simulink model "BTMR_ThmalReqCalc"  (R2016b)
settings: Solver=FixedStepDiscrete  StartTime=0.0  StopTime=10.0  FixedStep=0.1  RelTol=1e-3  EnableMultiTasking=on
undefined symbols (not defined in the file or in its folder): BMS_cntThmStbNum_C, BTMR_cntThmalReqVal_C, BTMR_flgCoolPwrCal_C, BTMR_pChrgClntPwrLv1_C, BTMR_pChrgClntPwrLv2_C, BTMR_pChrgClntPwrLv3_C, BTMR_pChrgClntPwrLv4_C, BTMR_pChrgClntPwrLv5_C, BTMR_pChrgClntPwrLv6_C, BTMR_pCoolPwrVal_C, BTMR_pHtgACPwrReq_C, BTMR_pHtgDCPwrReq_C, BTMR_pHtgDrvPwrReq_C, BTMR_pHtgsStage1_CUR, BTMR_pHtgsStage2_CUR, BTMR_pNormClntPwrLv1_C, BTMR_pNormClntPwrLv2_C, BTMR_pNormClntPwrLv3_C, BTMR_r861BrsDrvSoc_C, BTMR_r861HtgDrvSoc_C, BTMR_r891BrsDrvSoc_C, BTMR_r891HtgDrvSoc_C, BTMR_rCoolClbFlg_C, BTMR_rFlashClbFlg_C, BTMR_rHeatClbFlg_C, BTMR_t861BrsDiffLv0Temp_C, BTMR_t861BrsDiffLv1Temp_C, BTMR_t861CoolChrgAces2Temp_C, BTMR_t861CoolChrgAces3Temp_C, BTMR_t861CoolChrgAcesTemp_C, BTMR_t861CoolChrgDiffDebTemp_C, BTMR_t861CoolChrgEndDiffTemp_C, BTMR_t861CoolChrgExitLv2Temp_C, BTMR_t861CoolChrgExitLv3Temp_C, BTMR_t861CoolChrgExitTemp_C, BTMR_t861CoolChrgIntLv0Temp_C, BTMR_t861CoolChrgIntLv1Temp_C, BTMR_t861CoolChrgIntLv2Temp_C, BTMR_t861CoolChrgIntLv3Temp_C, BTMR_t861CoolChrgIntLv4Temp_C, BTMR_t861CoolChrgIntLv5Temp_C, BTMR_t861CoolDCDebTemp_C, BTMR_t861CoolNormAcesTemp_C, BTMR_t861CoolNormDiffDebTemp_C, BTMR_t861CoolNormEndDiffTemp_C, BTMR_t861CoolNormExitLv2Temp_C, BTMR_t861CoolNormExitLv3Temp_C, BTMR_t861CoolNormExitTemp_C, BTMR_t861CoolNormIntLv0Temp_C, BTMR_t861CoolNormIntLv1Temp_C, BTMR_t861CoolNormLv2Temp_C, BTMR_t861CoolNormLv3Temp_C, BTMR_t861HtgACDiffDebTemp_C, BTMR_t861HtgACEndDiffTemp_C, BTMR_t861HtgACStartHiTemp_C, BTMR_t861HtgACStartLoTemp_C, BTMR_t861HtgACStopTemp_C, BTMR_t861HtgDCDiffDebTemp_C, BTMR_t861HtgDCEndDiffTemp_C, BTMR_t861HtgDCIntLv0Temp_C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
libraries: AIWAYS_Powertrain_BMS_lib x78, simulink x9
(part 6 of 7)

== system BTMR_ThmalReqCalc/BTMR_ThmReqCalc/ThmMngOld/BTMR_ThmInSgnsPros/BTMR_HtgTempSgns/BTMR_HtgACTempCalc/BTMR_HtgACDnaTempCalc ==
  BSPR_tCellTempMin : Inport
  BMSDebounceStartZero : AIWAYS_Powertrain_BMS_lib/Debounce & Delay/BMSDebounceStartZero
  Constant29 : Constant  Value=BTMR_tiTempBase_C
  Constant30 : Constant  Value=BTMR_tiTempDebs_C
  Constant8 : Constant  Value=BTMR_t861HtgACStopTemp_C
  Relational Operator18 : RelationalOperator  OutDataTypeStr=boolean  RndMeth=Simplest
  BTMR_flgHtgACDnaTemp : Outport
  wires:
  Constant8/1 -> Relational Operator18/2
  BMSDebounceStartZero/1 -> BTMR_flgHtgACDnaTemp/1
  Relational Operator18/1 -> BMSDebounceStartZero/1
  BSPR_tCellTempMin/1 -> Relational Operator18/1
  Constant29/1 -> BMSDebounceStartZero/5, BMSDebounceStartZero/3
  Constant30/1 -> BMSDebounceStartZero/4, BMSDebounceStartZero/2

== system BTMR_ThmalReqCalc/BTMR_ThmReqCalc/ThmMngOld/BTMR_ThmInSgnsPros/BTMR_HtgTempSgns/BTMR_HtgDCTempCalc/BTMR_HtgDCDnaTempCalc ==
  BSPR_tCellTempMin : Inport
  BSPR_tCellTempMax : Inport  Port=2
  BMSDebounceStartZero : AIWAYS_Powertrain_BMS_lib/Debounce & Delay/BMSDebounceStartZero
  Constant1 : Constant  Value=BTMR_t861HtgDCStopTemp2_C
  Constant16 : Constant  Value=BTMR_t861HtgDCStopTemp_C
  Constant29 : Constant  Value=BTMR_tiTempBase_C
  Constant30 : Constant  Value=BTMR_tiTempDebs_C
  Logical Operator4 : Logic  Operator=OR  AllPortsSameDT=off  OutDataTypeStr=boolean
  Relational Operator1 : RelationalOperator  Operator=>  OutDataTypeStr=boolean  RndMeth=Simplest
  Relational Operator18 : RelationalOperator  Operator=>  OutDataTypeStr=boolean  RndMeth=Simplest
  BTMR_flgHtgDCDnaTemp : Outport
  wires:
  BSPR_tCellTempMin/1 -> Relational Operator18/1
  Relational Operator18/1 -> Logical Operator4/1
  BMSDebounceStartZero/1 -> BTMR_flgHtgDCDnaTemp/1
  Constant16/1 -> Relational Operator18/2
  BSPR_tCellTempMax/1 -> Relational Operator1/1
  Constant1/1 -> Relational Operator1/2
  Relational Operator1/1 -> Logical Operator4/2
  Logical Operator4/1 -> BMSDebounceStartZero/1
  Constant29/1 -> BMSDebounceStartZero/5, BMSDebounceStartZero/3
  Constant30/1 -> BMSDebounceStartZero/4, BMSDebounceStartZero/2

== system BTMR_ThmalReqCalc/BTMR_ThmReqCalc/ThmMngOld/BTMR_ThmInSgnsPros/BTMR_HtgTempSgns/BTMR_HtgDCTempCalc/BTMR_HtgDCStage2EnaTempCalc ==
  BSPR_tClntUsT : Inport
  BMSDebounceStartZero : AIWAYS_Powertrain_BMS_lib/Debounce & Delay/BMSDebounceStartZero
  Constant22 : Constant  Value=BTMR_t861HtgDCIntLv4Temp_C
  Constant29 : Constant  Value=BTMR_tiTempBase_C
  Constant30 : Constant  Value=BTMR_tiTempDebs_C
  Relational Operator20 : RelationalOperator  OutDataTypeStr=boolean  RndMeth=Simplest
  BTMR_flgHtgDCStage2EnaTemp : Outport
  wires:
  BSPR_tClntUsT/1 -> Relational Operator20/1
  BMSDebounceStartZero/1 -> BTMR_flgHtgDCStage2EnaTemp/1
  Relational Operator20/1 -> BMSDebounceStartZero/1
  Constant22/1 -> Relational Operator20/2
  Constant29/1 -> BMSDebounceStartZero/5, BMSDebounceStartZero/3
  Constant30/1 -> BMSDebounceStartZero/4, BMSDebounceStartZero/2

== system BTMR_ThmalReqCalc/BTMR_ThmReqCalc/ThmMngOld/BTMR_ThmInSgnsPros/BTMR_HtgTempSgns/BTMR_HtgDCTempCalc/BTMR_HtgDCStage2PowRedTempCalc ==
  BSPR_tClntUsT : Inport
  BMSDebounceStartZero : AIWAYS_Powertrain_BMS_lib/Debounce & Delay/BMSDebounceStartZero
  Constant22 : Constant  Value=BTMR_t861HtgDCIntLv3Temp_C
  Constant29 : Constant  Value=BTMR_tiTempBase_C
  Constant30 : Constant  Value=BTMR_tiTempDebs_C
  Relational Operator20 : RelationalOperator  OutDataTypeStr=boolean  RndMeth=Simplest
  BTMR_flgHtgDCStage2PowRedTemp : Outport
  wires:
  Constant22/1 -> Relational Operator20/2
  Relational Operator20/1 -> BMSDebounceStartZero/1
  BMSDebounceStartZero/1 -> BTMR_flgHtgDCStage2PowRedTemp/1
  BSPR_tClntUsT/1 -> Relational Operator20/1
  Constant29/1 -> BMSDebounceStartZero/5, BMSDebounceStartZero/3
  Constant30/1 -> BMSDebounceStartZero/4, BMSDebounceStartZero/2

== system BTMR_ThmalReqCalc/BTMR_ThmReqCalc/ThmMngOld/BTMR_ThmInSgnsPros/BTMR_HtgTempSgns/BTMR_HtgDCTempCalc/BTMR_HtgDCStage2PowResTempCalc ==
  BSPR_tClntUsT : Inport
  BMSDebounceStartZero : AIWAYS_Powertrain_BMS_lib/Debounce & Delay/BMSDebounceStartZero
  Constant22 : Constant  Value=BTMR_t861HtgDCIntLv2Temp_C
  Constant29 : Constant  Value=BTMR_tiTempBase_C
  Constant30 : Constant  Value=BTMR_tiTempDebs_C
  Relational Operator20 : RelationalOperator  Operator=<=  OutDataTypeStr=boolean  RndMeth=Simplest
  BTMR_flgHtgDCStage2PowResTemp : Outport
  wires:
  BSPR_tClntUsT/1 -> Relational Operator20/1
  BMSDebounceStartZero/1 -> BTMR_flgHtgDCStage2PowResTemp/1
  Relational Operator20/1 -> BMSDebounceStartZero/1
  Constant22/1 -> Relational Operator20/2
  Constant29/1 -> BMSDebounceStartZero/5, BMSDebounceStartZero/3
  Constant30/1 -> BMSDebounceStartZero/4, BMSDebounceStartZero/2

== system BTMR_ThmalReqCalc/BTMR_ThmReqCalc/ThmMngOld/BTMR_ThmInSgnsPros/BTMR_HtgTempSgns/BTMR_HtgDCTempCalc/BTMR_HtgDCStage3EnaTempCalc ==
  BSPR_tCellTempMin : Inport
  BSPR_tCellTempMax : Inport  Port=2
  BMSDebounceStartZero : AIWAYS_Powertrain_BMS_lib/Debounce & Delay/BMSDebounceStartZero
  Constant23 : Constant  Value=BTMR_t861HtgDCStageMxTemp_C
  Constant24 : Constant  Value=BTMR_t861HtgDCStageMnTemp_C
  Constant29 : Constant  Value=BTMR_tiTempBase_C
  Constant30 : Constant  Value=BTMR_tiTempDebs_C
  Logical Operator1 : Logic  Operator=NOT  AllPortsSameDT=off  OutDataTypeStr=boolean
  Logical Operator4 : Logic  AllPortsSameDT=off  OutDataTypeStr=boolean
  Relational Operator12 : RelationalOperator  Operator=<  OutDataTypeStr=boolean  RndMeth=Simplest
  Relational Operator13 : RelationalOperator  Operator=<  OutDataTypeStr=boolean  RndMeth=Simplest
  BTMR_flgHtgDCStage3EnaTemp : Outport
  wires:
  BSPR_tCellTempMin/1 -> Relational Operator12/1
  Logical Operator4/1 -> Logical Operator1/1
  Constant24/1 -> Relational Operator12/2
  Relational Operator13/1 -> Logical Operator4/2
  Constant23/1 -> Relational Operator13/2
  Relational Operator12/1 -> Logical Operator4/1
  BMSDebounceStartZero/1 -> BTMR_flgHtgDCStage3EnaTemp/1
  BSPR_tCellTempMax/1 -> Relational Operator13/1
  Logical Operator1/1 -> BMSDebounceStartZero/1
  Constant29/1 -> BMSDebounceStartZero/5, BMSDebounceStartZero/3
  Constant30/1 -> BMSDebounceStartZero/4, BMSDebounceStartZero/2

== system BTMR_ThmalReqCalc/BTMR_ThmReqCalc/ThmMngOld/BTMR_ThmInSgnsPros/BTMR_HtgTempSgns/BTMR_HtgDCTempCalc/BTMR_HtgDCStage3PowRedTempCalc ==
  BSPR_tClntUsT : Inport
  BMSDebounceStartZero : AIWAYS_Powertrain_BMS_lib/Debounce & Delay/BMSDebounceStartZero
  Constant22 : Constant  Value=BTMR_t861HtgDCIntLv1Temp_C
  Constant29 : Constant  Value=BTMR_tiTempBase_C
  Constant30 : Constant  Value=BTMR_tiTempDebs_C
  Relational Operator20 : RelationalOperator  Operator=<=  OutDataTypeStr=boolean  RndMeth=Simplest
  BTMR_flgHtgDCStage3PowRedTemp : Outport
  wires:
  BSPR_tClntUsT/1 -> Relational Operator20/1
  BMSDebounceStartZero/1 -> BTMR_flgHtgDCStage3PowRedTemp/1
  Relational Operator20/1 -> BMSDebounceStartZero/1
  Constant22/1 -> Relational Operator20/2
  Constant29/1 -> BMSDebounceStartZero/5, BMSDebounceStartZero/3
  Constant30/1 -> BMSDebounceStartZero/4, BMSDebounceStartZero/2

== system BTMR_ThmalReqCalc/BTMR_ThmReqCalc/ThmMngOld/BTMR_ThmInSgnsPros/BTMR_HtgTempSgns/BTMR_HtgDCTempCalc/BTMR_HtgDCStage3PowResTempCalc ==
  BSPR_tClntUsT : Inport
  BMSDebounceStartZero : AIWAYS_Powertrain_BMS_lib/Debounce & Delay/BMSDebounceStartZero
  Constant22 : Constant  Value=BTMR_t861HtgDCIntLv0Temp_C
  Constant29 : Constant  Value=BTMR_tiTempBase_C
  Constant30 : Constant  Value=BTMR_tiTempDebs_C
  Relational Operator20 : RelationalOperator  Operator=<=  OutDataTypeStr=boolean  RndMeth=Simplest
  BTMR_flgHtgDCStage3PowResTemp : Outport
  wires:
  Constant22/1 -> Relational Operator20/2
  Relational Operator20/1 -> BMSDebounceStartZero/1
  BMSDebounceStartZero/1 -> BTMR_flgHtgDCStage3PowResTemp/1
  BSPR_tClntUsT/1 -> Relational Operator20/1
  Constant29/1 -> BMSDebounceStartZero/5, BMSDebounceStartZero/3
  Constant30/1 -> BMSDebounceStartZero/4, BMSDebounceStartZero/2

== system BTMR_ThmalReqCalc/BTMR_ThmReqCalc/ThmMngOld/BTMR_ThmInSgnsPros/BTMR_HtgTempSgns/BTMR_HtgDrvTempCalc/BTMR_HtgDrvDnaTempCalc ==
  BSPR_tCellTempMin : Inport
  BMSDebounceStartZero : AIWAYS_Powertrain_BMS_lib/Debounce & Delay/BMSDebounceStartZero
  Constant2 : Constant  Value=BTMR_t861HtgDrvStopTemp_C
  Constant29 : Constant  Value=BTMR_tiTempBase_C
  Constant30 : Constant  Value=BTMR_tiTempDebs_C
  Relational Operator18 : RelationalOperator  OutDataTypeStr=boolean  RndMeth=Simplest
  BTMR_flgHtgDrvDnaTemp : Outport
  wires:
  BSPR_tCellTempMin/1 -> Relational Operator18/1
  Relational Operator18/1 -> BMSDebounceStartZero/1
  BMSDebounceStartZero/1 -> BTMR_flgHtgDrvDnaTemp/1
  Constant2/1 -> Relational Operator18/2
  Constant29/1 -> BMSDebounceStartZero/5, BMSDebounceStartZero/3
  Constant30/1 -> BMSDebounceStartZero/4, BMSDebounceStartZero/2

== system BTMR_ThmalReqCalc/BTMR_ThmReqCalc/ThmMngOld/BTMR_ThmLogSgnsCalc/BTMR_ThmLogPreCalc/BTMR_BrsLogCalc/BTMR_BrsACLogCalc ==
  BTMR_flgBMSStsSgns : Inport
  BTMR_flgBrsEnSgns : Inport  Port=2
  BTMR_flgBrsIntSgns : Inport  Port=3
  Bus Creator : BusCreator  Inputs=3
  Bus Selector : BusSelector  OutputSignals=BTMR_flgBMSAChrg
  Bus Selector2 : BusSelector  OutputSignals=BTMR_flgBrsEna2Temp
  Bus Selector3 : BusSelector  OutputSignals=BTMR_flgBrsIntEna2Temp
  Logical Operator1 : Logic  Operator=NOT  AllPortsSameDT=off  OutDataTypeStr=boolean
  Logical Operator{2..4,6} (4 alike) : Logic  AllPortsSameDT=off  OutDataTypeStr=boolean
  Logical Operator5 : Logic  Operator=NOT  AllPortsSameDT=off  OutDataTypeStr=boolean
  BTMR_flgBrsACLogSgns : Outport
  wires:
  Bus Selector3/1 -> Logical Operator5/1, Logical Operator3/2  "<BTMR_flgBrsIntEna2Temp>"
  Logical Operator6/1 -> Logical Operator3/1, Logical Operator4/1  "BTMR_flgBrsEna2"
  Logical Operator2/1 -> Bus Creator/2  "BTMR_flgBrsACOut"
  Logical Operator1/1 -> Logical Operator2/2
  Bus Selector/1 -> Logical Operator2/1, Logical Operator6/1  "<BTMR_flgBMSAChrg>"
  BTMR_flgBrsEnSgns/1 -> Bus Selector2/1
  BTMR_flgBrsIntSgns/1 -> Bus Selector3/1
  BTMR_flgBMSStsSgns/1 -> Bus Selector/1
  Logical Operator4/1 -> Bus Creator/3  "BTMR_flgBrsACout2"
  Bus Selector2/1 -> Logical Operator1/1, Logical Operator6/2  "<BTMR_flgBrsEna2Temp>"
  Logical Operator3/1 -> Bus Creator/1  "BTMR_flgBrsIntEna2"
  Logical Operator5/1 -> Logical Operator4/2
  Bus Creator/1 -> BTMR_flgBrsACLogSgns/1  "BTMR_flgBrsACLogSgns"

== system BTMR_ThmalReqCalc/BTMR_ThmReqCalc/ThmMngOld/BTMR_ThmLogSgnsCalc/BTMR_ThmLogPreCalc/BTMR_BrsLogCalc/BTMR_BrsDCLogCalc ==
  BTMR_flgBMSStsSgns : Inport
  BTMR_flgBrsEnSgns : Inport  Port=2
  BTMR_flgBrsIntSgns : Inport  Port=3
  Bus Creator : BusCreator  Inputs=3
  Bus Selector : BusSelector  OutputSignals=BTMR_flgBMSDChrg
  Bus Selector2 : BusSelector  OutputSignals=BTMR_flgBrsEna1Temp
  Bus Selector3 : BusSelector  OutputSignals=BTMR_flgBrsIntEna1Temp
  Logical Operator1 : Logic  Operator=NOT  AllPortsSameDT=off  OutDataTypeStr=boolean
  Logical Operator{2..4,6} (4 alike) : Logic  AllPortsSameDT=off  OutDataTypeStr=boolean
  Logical Operator5 : Logic  Operator=NOT  AllPortsSameDT=off  OutDataTypeStr=boolean
  BTMR_flgBrsDCLogSgns : Outport
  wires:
  Bus Creator/1 -> BTMR_flgBrsDCLogSgns/1  "BTMR_flgBrsDCLogSgns"
  Logical Operator5/1 -> Logical Operator4/2
  Logical Operator3/1 -> Bus Creator/1  "BTMR_flgBrsIntEna1"
  Bus Selector2/1 -> Logical Operator6/2, Logical Operator1/1  "<BTMR_flgBrsEna1Temp>"
  Logical Operator4/1 -> Bus Creator/3  "BTMR_flgBrsDCout2"
  BTMR_flgBMSStsSgns/1 -> Bus Selector/1
  BTMR_flgBrsIntSgns/1 -> Bus Selector3/1
  BTMR_flgBrsEnSgns/1 -> Bus Selector2/1
  Bus Selector/1 -> Logical Operator6/1, Logical Operator2/1  "<BTMR_flgBMSDChrg>"
  Logical Operator1/1 -> Logical Operator2/2
  Logical Operator2/1 -> Bus Creator/2  "BTMR_flgBrsDCOut"
  Logical Operator6/1 -> Logical Operator3/1, Logical Operator4/1  "BTMR_flgBrsEna1"
  Bus Selector3/1 -> Logical Operator3/2, Logical Operator5/1  "<BTMR_flgBrsIntEna1Temp>"

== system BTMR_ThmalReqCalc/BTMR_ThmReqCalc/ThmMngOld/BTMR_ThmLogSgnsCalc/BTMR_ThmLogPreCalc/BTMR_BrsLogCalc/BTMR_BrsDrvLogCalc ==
  BTMR_flgBMSStsSgns : Inport
  BTMR_flgBrsEnSgns : Inport  Port=2
  BTMR_flgBrsIntSgns : Inport  Port=3
  BTMR_flgSOCSgns : Inport  Port=4
  Bus Creator : BusCreator  Inputs=4
  Bus Selector : BusSelector  OutputSignals=BTMR_flgBMSDrv
  Bus Selector1 : BusSelector  OutputSignals=BTMR_flgBrsDrvSOC
  Bus Selector2 : BusSelector  OutputSignals=BTMR_flgBrsEna3Temp
  Bus Selector3 : BusSelector  OutputSignals=BTMR_flgBrsIntEna3Temp
  Logical Operator1 : Logic  Operator=NOT  AllPortsSameDT=off  OutDataTypeStr=boolean
  Logical Operator{2..4,6..7,9} (6 alike) : Logic  AllPortsSameDT=off  OutDataTypeStr=boolean
  Logical Operator5 : Logic  Operator=NOT  AllPortsSameDT=off  OutDataTypeStr=boolean
  Logical Operator8 : Logic  Operator=NOT  AllPortsSameDT=off  OutDataTypeStr=boolean
  BTMR_flgBrsDrvLogSgns : Outport
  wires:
  Bus Creator/1 -> BTMR_flgBrsDrvLogSgns/1  "BTMR_flgBrsDrvLogSgns"
  Logical Operator5/1 -> Logical Operator4/2
  Logical Operator7/1 -> Bus Creator/1  "BTMR_flgBrsIntEna3"
  Bus Selector2/1 -> Logical Operator1/1, Logical Operator6/2  "<BTMR_flgBrsEna3Temp>"
  Logical Operator9/1 -> Bus Creator/3  "BTMR_flgBrsDrvOut2"
  BTMR_flgBMSStsSgns/1 -> Bus Selector/1
  BTMR_flgBrsIntSgns/1 -> Bus Selector3/1
  BTMR_flgBrsEnSgns/1 -> Bus Selector2/1
  Bus Selector/1 -> Logical Operator6/1, Logical Operator2/1  "<BTMR_flgBMSDrv>"
  Logical Operator1/1 -> Logical Operator2/2
  Logical Operator6/1 -> Logical Operator9/1, Logical Operator3/1  "BTMR_flgBrsEna3"
  Bus Selector3/1 -> Logical Operator5/1, Logical Operator7/2  "<BTMR_flgBrsIntEna3Temp>"
  BTMR_flgSOCSgns/1 -> Bus Selector1/1
  Bus Selector1/1 -> Logical Operator3/2, Logical Operator8/1  "<BTMR_flgBrsDrvSOC>"
  Logical Operator3/1 -> Logical Operator4/1, Logical Operator7/1  "BTMR_flgBrsSOCEna3"
  Logical Operator2/1 -> Bus Creator/2  "BTMR_flgBrsDrvOut"
  Logical Operator8/1 -> Logical Operator9/2
  Logical Operator4/1 -> Bus Creator/4  "BTMR_flgBrsDrvOut3"

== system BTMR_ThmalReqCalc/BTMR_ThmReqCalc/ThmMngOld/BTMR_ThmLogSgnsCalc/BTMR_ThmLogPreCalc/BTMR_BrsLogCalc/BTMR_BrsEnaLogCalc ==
  BTMR_flgBrsDCLogSgns : Inport
  BTMR_flgBrsACLogSgns : Inport  Port=2
  BTMR_flgBrsDrvLogSgns : Inport  Port=3
  BTMR_flgBrsTempSgns : Inport  Port=4
  BTMR_BrsEnaCalc : Subsystem
  Bus Creator : BusCreator  Inputs=3
  Bus Creator2 : BusCreator  Inputs=2
  Bus Selector : BusSelector  OutputSignals=BTMR_flgBrsInTempSgns
  Bus Selector2 : BusSelector  OutputSignals=BTMR_flgBrsStartTemp
  Logical Operator1 : Logic  Operator=NOT  AllPortsSameDT=off  OutDataTypeStr=boolean
  Logical Operator3 : Logic  AllPortsSameDT=off  OutDataTypeStr=boolean
  BTMR_flgBrsEnaLogSgns : Outport
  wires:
  BTMR_flgBrsDCLogSgns/1 -> Bus Creator/1
  BTMR_flgBrsACLogSgns/1 -> Bus Creator/2
  BTMR_flgBrsDrvLogSgns/1 -> Bus Creator/3
  Bus Creator/1 -> BTMR_BrsEnaCalc/1(BTMR_flgBrsInLogSgns)  "BTMR_flgBrsInLogSgns"
  Bus Selector/1 -> Bus Selector2/1  "<BTMR_flgBrsInTempSgns>"
  Bus Selector2/1 -> Logical Operator1/1  "<BTMR_flgBrsStartTemp>"
  BTMR_BrsEnaCalc/1(BTMR_flgBrsEna) -> Logical Operator3/1, Bus Creator2/1  "BTMR_flgBrsEna"
  Logical Operator1/1 -> Logical Operator3/2
  Logical Operator3/1 -> Bus Creator2/2  "BTMR_flgBrsOut"
  BTMR_flgBrsTempSgns/1 -> Bus Selector/1
  Bus Creator2/1 -> BTMR_flgBrsEnaLogSgns/1  "BTMR_flgBrsEnaLogSgns"

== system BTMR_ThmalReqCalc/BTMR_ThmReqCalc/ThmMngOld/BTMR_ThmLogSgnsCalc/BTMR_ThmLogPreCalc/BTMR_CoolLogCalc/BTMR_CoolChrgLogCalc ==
  BTMR_flgHtgLogSgns : Inport
  BTMR_flgThmEnaTempSgns : Inport  Port=2
  Bus Creator : BusCreator  Inputs=2
  Bus Selector : BusSelector  OutputSignals=BTMR_flgHtgDCLogSgns
  Bus Selector1 : BusSelector  OutputSignals=BTMR_flgHtgDCOut
  Bus Selector2 : BusSelector  OutputSignals=BTMR_CoolChrgEnaTemp
  Logical Operator1 : Logic  Operator=NOT  AllPortsSameDT=off  OutDataTypeStr=boolean
  Logical Operator2 : Logic  AllPortsSameDT=off  OutDataTypeStr=boolean
  Logical Operator3 : Logic  AllPortsSameDT=off  OutDataTypeStr=boolean
  BTMR_flgCoolChrgLogSgns : Outport
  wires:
  Bus Creator/1 -> BTMR_flgCoolChrgLogSgns/1  "BTMR_flgCoolChrgLogSgns"
  BTMR_flgThmEnaTempSgns/1 -> Bus Selector2/1
  Bus Selector1/1 -> Logical Operator3/1, Logical Operator2/1  "<BTMR_flgHtgDCOut>"
  Bus Selector2/1 -> Logical Operator1/1, Logical Operator3/2  "<BTMR_CoolChrgEnaTemp>"
  Logical Operator1/1 -> Logical Operator2/2
  Logical Operator3/1 -> Bus Creator/1  "BTMR_flgCoolChrgEna"
  Logical Operator2/1 -> Bus Creator/2  "BTMR_flgCoolChrgOut"
  Bus Selector/1 -> Bus Selector1/1  "<BTMR_flgHtgDCLogSgns>"
  BTMR_flgHtgLogSgns/1 -> Bus Selector/1

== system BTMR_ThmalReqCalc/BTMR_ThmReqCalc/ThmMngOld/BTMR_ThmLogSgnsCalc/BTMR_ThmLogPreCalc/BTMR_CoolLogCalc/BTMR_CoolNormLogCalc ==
  BTMR_flgHtgLogSgns : Inport
  BTMR_flgThmEnaTempSgns : Inport  Port=2
  Bus Creator : BusCreator  Inputs=2
  Bus Selector : BusSelector  OutputSignals=BTMR_flgHtgACLogSgns,BTMR_flgHtgDrvLogSgns
  Bus Selector1 : BusSelector  OutputSignals=BTMR_flgHtgACOut
  Bus Selector2 : BusSelector  OutputSignals=BTMR_CoolNormEnaTemp
  Bus Selector3 : BusSelector  OutputSignals=BTMR_flgHtgDrvOut
  Logical Operator1 : Logic  Operator=NOT  AllPortsSameDT=off  OutDataTypeStr=boolean
  Logical Operator2 : Logic  AllPortsSameDT=off  OutDataTypeStr=boolean
  Logical Operator3 : Logic  AllPortsSameDT=off  OutDataTypeStr=boolean
  Logical Operator4 : Logic  Operator=OR  AllPortsSameDT=off  OutDataTypeStr=boolean
  BTMR_flgCoolNormLogSgns : Outport
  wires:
  BTMR_flgHtgLogSgns/1 -> Bus Selector/1
  Bus Selector/1 -> Bus Selector1/1  "<BTMR_flgHtgACLogSgns>"
  Logical Operator2/1 -> Bus Creator/2  "BTMR_flgCoolNormOut"
  Logical Operator3/1 -> Bus Creator/1  "BTMR_flgCoolNormEna"
  Logical Operator1/1 -> Logical Operator2/2
  Bus Selector2/1 -> Logical Operator3/2, Logical Operator1/1  "<BTMR_CoolNormEnaTemp>"
  Logical Operator4/1 -> Logical Operator2/1, Logical Operator3/1
  BTMR_flgThmEnaTempSgns/1 -> Bus Selector2/1
  Bus Creator/1 -> BTMR_flgCoolNormLogSgns/1  "BTMR_flgCoolNormLogSgns"
  Bus Selector/2 -> Bus Selector3/1  "<BTMR_flgHtgDrvLogSgns>"
  Bus Selector1/1 -> Logical Operator4/1  "<BTMR_flgHtgACOut>"
  Bus Selector3/1 -> Logical Operator4/2  "<BTMR_flgHtgDrvOut>"

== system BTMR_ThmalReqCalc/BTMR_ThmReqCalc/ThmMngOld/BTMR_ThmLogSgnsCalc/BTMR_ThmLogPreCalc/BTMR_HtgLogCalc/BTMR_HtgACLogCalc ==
  BTMR_flgBrsLogSgns : Inport
  BTMR_flgThmEnaTempSgns : Inport  Port=2
  Bus Creator : BusCreator  Inputs=2
  Bus Selector : BusSelector  OutputSignals=BTMR_flgBrsACLogSgns
  Bus Selector1 : BusSelector  OutputSignals=BTMR_flgBrsACOut
  Bus Selector2 : BusSelector  OutputSignals=BTMR_HtgACEnaTemp
  Logical Operator1 : Logic  Operator=NOT  AllPortsSameDT=off  OutDataTypeStr=boolean
  Logical Operator2 : Logic  AllPortsSameDT=off  OutDataTypeStr=boolean
  Logical Operator3 : Logic  AllPortsSameDT=off  OutDataTypeStr=boolean
  BTMR_flgHtgACLogSgns : Outport
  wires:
  Bus Creator/1 -> BTMR_flgHtgACLogSgns/1  "BTMR_flgHtgACLogSgns"
  BTMR_flgThmEnaTempSgns/1 -> Bus Selector2/1
  Bus Selector1/1 -> Logical Operator3/1, Logical Operator2/1  "<BTMR_flgBrsACOut>"
  Bus Selector2/1 -> Logical Operator1/1, Logical Operator3/2  "<BTMR_HtgACEnaTemp>"
  Logical Operator1/1 -> Logical Operator2/2
  Logical Operator3/1 -> Bus Creator/1  "BTMR_flgHtgACEna"
  Logical Operator2/1 -> Bus Creator/2  "BTMR_flgHtgACOut"
  Bus Selector/1 -> Bus Selector1/1  "<BTMR_flgBrsACLogSgns>"
  BTMR_flgBrsLogSgns/1 -> Bus Selector/1

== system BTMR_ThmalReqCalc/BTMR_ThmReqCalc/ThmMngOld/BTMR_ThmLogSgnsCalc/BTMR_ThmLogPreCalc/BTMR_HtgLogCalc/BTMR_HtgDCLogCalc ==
  BTMR_flgBrsLogSgns : Inport
  BTMR_flgThmEnaTempSgns : Inport  Port=2
  Bus Creator : BusCreator  Inputs=2
  Bus Selector : BusSelector  OutputSignals=BTMR_flgBrsDCLogSgns
  Bus Selector1 : BusSelector  OutputSignals=BTMR_flgBrsDCOut
  Bus Selector2 : BusSelector  OutputSignals=BTMR_HtgDCEnaTemp
  Logical Operator1 : Logic  Operator=NOT  AllPortsSameDT=off  OutDataTypeStr=boolean
  Logical Operator2 : Logic  AllPortsSameDT=off  OutDataTypeStr=boolean
  Logical Operator3 : Logic  AllPortsSameDT=off  OutDataTypeStr=boolean
  BTMR_flgHtgDCLogSgns : Outport
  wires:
  BTMR_flgBrsLogSgns/1 -> Bus Selector/1
  Bus Selector/1 -> Bus Selector1/1  "<BTMR_flgBrsDCLogSgns>"
  Logical Operator2/1 -> Bus Creator/2  "BTMR_flgHtgDCOut"
  Logical Operator3/1 -> Bus Creator/1  "BTMR_flgHtgDCEna"
  Logical Operator1/1 -> Logical Operator2/2
  Bus Selector2/1 -> Logical Operator3/2, Logical Operator1/1  "<BTMR_HtgDCEnaTemp>"
  Bus Selector1/1 -> Logical Operator2/1, Logical Operator3/1  "<BTMR_flgBrsDCOut>"
  BTMR_flgThmEnaTempSgns/1 -> Bus Selector2/1
  Bus Creator/1 -> BTMR_flgHtgDCLogSgns/1  "BTMR_flgHtgDCLogSgns"

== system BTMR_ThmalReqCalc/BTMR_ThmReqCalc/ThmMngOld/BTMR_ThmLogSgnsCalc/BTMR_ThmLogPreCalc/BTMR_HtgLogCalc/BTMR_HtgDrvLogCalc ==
  BTMR_flgBrsLogSgns : Inport
  BTMR_flgThmEnaTempSgns : Inport  Port=2
  Bus Creator : BusCreator  Inputs=2
  Bus Selector : BusSelector  OutputSignals=BTMR_flgBrsDrvLogSgns
  Bus Selector1 : BusSelector  OutputSignals=BTMR_flgBrsDrvOut
  Bus Selector2 : BusSelector  OutputSignals=BTMR_HtgDrvEnaTemp
  Logical Operator1 : Logic  Operator=NOT  AllPortsSameDT=off  OutDataTypeStr=boolean
  Logical Operator2 : Logic  AllPortsSameDT=off  OutDataTypeStr=boolean
  Logical Operator3 : Logic  AllPortsSameDT=off  OutDataTypeStr=boolean
  BTMR_flgHtgDrvLogSgns : Outport
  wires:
  BTMR_flgBrsLogSgns/1 -> Bus Selector/1
  Bus Selector/1 -> Bus Selector1/1  "<BTMR_flgBrsDrvLogSgns>"
  Logical Operator2/1 -> Bus Creator/2  "BTMR_flgHtgDrvOut"
  Logical Operator1/1 -> Logical Operator2/2
  Bus Selector2/1 -> Logical Operator3/2, Logical Operator1/1  "<BTMR_HtgDrvEnaTemp>"
  Bus Selector1/1 -> Logical Operator2/1, Logical Operator3/1  "<BTMR_flgBrsDrvOut>"
  BTMR_flgThmEnaTempSgns/1 -> Bus Selector2/1
  Bus Creator/1 -> BTMR_flgHtgDrvLogSgns/1  "BTMR_flgHtgDrvLogSgns"
  Logical Operator3/1 -> Bus Creator/1  "BTMR_flgHtgDrvEna"

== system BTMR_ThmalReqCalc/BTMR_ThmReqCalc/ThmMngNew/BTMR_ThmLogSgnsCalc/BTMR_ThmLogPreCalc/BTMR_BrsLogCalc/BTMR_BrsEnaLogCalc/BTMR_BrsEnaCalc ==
  BTMR_flgBrsInLogSgns : Inport
  Bus Selector : BusSelector  OutputSignals=BTMR_flgBrsDCLogSgns,BTMR_flgBrsACLogSgns,BTMR_flgBrsDrvLogSgns
  Bus Selector1 : BusSelector  OutputSignals=BTMR_flgBrsIntEna1
  Bus Selector2 : BusSelector  OutputSignals=BTMR_flgBrsIntEna2
  Bus Selector3 : BusSelector  OutputSignals=BTMR_flgBrsIntEna3
  Logical Operator3 : Logic  Operator=OR  Inputs=3  AllPortsSameDT=off  OutDataTypeStr=boolean
  BTMR_flgBrsEna : Outport
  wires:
  BTMR_flgBrsInLogSgns/1 -> Bus Selector/1
  Bus Selector/1 -> Bus Selector1/1  "<BTMR_flgBrsDCLogSgns>"
  Bus Selector/3 -> Bus Selector3/1  "<BTMR_flgBrsDrvLogSgns>"
  Logical Operator3/1 -> BTMR_flgBrsEna/1  "BTMR_flgBrsEna"
  Bus Selector1/1 -> Logical Operator3/1  "<BTMR_flgBrsIntEna1>"
  Bus Selector3/1 -> Logical Operator3/3  "<BTMR_flgBrsIntEna3>"
  Bus Selector2/1 -> Logical Operator3/2  "<BTMR_flgBrsIntEna2>"
  Bus Selector/2 -> Bus Selector2/1  "<BTMR_flgBrsACLogSgns>"

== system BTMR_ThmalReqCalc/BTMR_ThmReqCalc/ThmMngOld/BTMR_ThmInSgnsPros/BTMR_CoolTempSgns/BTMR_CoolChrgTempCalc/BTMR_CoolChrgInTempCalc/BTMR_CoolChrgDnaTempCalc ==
  BSPR_tCellTempMax : Inport
  BMSDebounceStartZero : AIWAYS_Powertrain_BMS_lib/Debounce & Delay/BMSDebounceStartZero
  Constant14 : Constant  Value=BTMR_t861CoolChrgExitTemp_C
  Constant29 : Constant  Value=BTMR_tiTempBase_C
  Constant30 : Constant  Value=BTMR_tiTempDebs_C
  Relational Operator20 : RelationalOperator  Operator=<=  OutDataTypeStr=boolean  RndMeth=Simplest
  BTMR_flgCoolChrgDnaTemp : Outport
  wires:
  Relational Operator20/1 -> BMSDebounceStartZero/1
  BMSDebounceStartZero/1 -> BTMR_flgCoolChrgDnaTemp/1
  BSPR_tCellTempMax/1 -> Relational Operator20/1
  Constant14/1 -> Relational Operator20/2
  Constant29/1 -> BMSDebounceStartZero/5, BMSDebounceStartZero/3
  Constant30/1 -> BMSDebounceStartZero/4, BMSDebounceStartZero/2

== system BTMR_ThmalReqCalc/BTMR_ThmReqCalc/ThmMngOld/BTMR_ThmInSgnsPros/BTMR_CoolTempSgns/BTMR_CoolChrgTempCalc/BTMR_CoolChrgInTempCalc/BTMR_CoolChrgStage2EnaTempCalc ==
  BSPR_tCellTempMax : Inport
  BMSDebounceStartZero : AIWAYS_Powertrain_BMS_lib/Debounce & Delay/BMSDebounceStartZero
  Constant15 : Constant  Value=BTMR_t861CoolChrgAces2Temp_C
  Constant29 : Constant  Value=BTMR_tiTempBase_C
  Constant30 : Constant  Value=BTMR_tiTempDebs_C
  Relational Operator20 : RelationalOperator  OutDataTypeStr=boolean  RndMeth=Simplest
  BTMR_flgCoolChrgStage2EnaTemp : Outport
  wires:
  Relational Operator20/1 -> BMSDebounceStartZero/1
  BMSDebounceStartZero/1 -> BTMR_flgCoolChrgStage2EnaTemp/1
  BSPR_tCellTempMax/1 -> Relational Operator20/1
  Constant15/1 -> Relational Operator20/2
  Constant29/1 -> BMSDebounceStartZero/5, BMSDebounceStartZero/3
  Constant30/1 -> BMSDebounceStartZero/4, BMSDebounceStartZero/2

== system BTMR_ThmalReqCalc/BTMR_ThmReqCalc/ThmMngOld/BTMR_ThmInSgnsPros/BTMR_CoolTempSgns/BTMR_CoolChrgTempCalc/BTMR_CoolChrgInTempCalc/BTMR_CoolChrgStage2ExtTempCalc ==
  BSPR_tCellTempMax : Inport
  BMSDebounceStartZero : AIWAYS_Powertrain_BMS_lib/Debounce & Delay/BMSDebounceStartZero
  Constant13 : Constant  Value=BTMR_t861CoolChrgExitLv2Temp_C
  Constant29 : Constant  Value=BTMR_tiTempBase_C
  Constant30 : Constant  Value=BTMR_tiTempDebs_C
  Relational Operator20 : RelationalOperator  Operator=<=  OutDataTypeStr=boolean  RndMeth=Simplest
  BTMR_flgCoolChrgStage2ExtTemp : Outport
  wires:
  Constant13/1 -> Relational Operator20/2
  BSPR_tCellTempMax/1 -> Relational Operator20/1
  BMSDebounceStartZero/1 -> BTMR_flgCoolChrgStage2ExtTemp/1
  Relational Operator20/1 -> BMSDebounceStartZero/1
  Constant29/1 -> BMSDebounceStartZero/5, BMSDebounceStartZero/3
  Constant30/1 -> BMSDebounceStartZero/4, BMSDebounceStartZero/2

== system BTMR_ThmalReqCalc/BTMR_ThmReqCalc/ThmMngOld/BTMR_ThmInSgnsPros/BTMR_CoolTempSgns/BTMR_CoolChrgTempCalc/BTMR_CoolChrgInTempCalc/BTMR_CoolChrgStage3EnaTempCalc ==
  BSPR_tCellTempMax : Inport
  BMSDebounceStartZero : AIWAYS_Powertrain_BMS_lib/Debounce & Delay/BMSDebounceStartZero
  Constant13 : Constant  Value=BTMR_t861CoolChrgAces3Temp_C
  Constant29 : Constant  Value=BTMR_tiTempBase_C
  Constant30 : Constant  Value=BTMR_tiTempDebs_C
  Relational Operator20 : RelationalOperator  OutDataTypeStr=boolean  RndMeth=Simplest
  BTMR_flgCoolChrgStage3EnaTemp : Outport
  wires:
  Constant13/1 -> Relational Operator20/2
  BSPR_tCellTempMax/1 -> Relational Operator20/1
  BMSDebounceStartZero/1 -> BTMR_flgCoolChrgStage3EnaTemp/1
  Relational Operator20/1 -> BMSDebounceStartZero/1
  Constant29/1 -> BMSDebounceStartZero/5, BMSDebounceStartZero/3
  Constant30/1 -> BMSDebounceStartZero/4, BMSDebounceStartZero/2

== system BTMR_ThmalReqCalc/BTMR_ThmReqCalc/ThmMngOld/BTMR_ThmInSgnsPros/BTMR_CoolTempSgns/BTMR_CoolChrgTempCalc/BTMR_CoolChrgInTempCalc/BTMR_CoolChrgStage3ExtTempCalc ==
  BSPR_tCellTempMax : Inport
  BMSDebounceStartZero : AIWAYS_Powertrain_BMS_lib/Debounce & Delay/BMSDebounceStartZero
  Constant13 : Constant  Value=BTMR_t861CoolChrgExitLv3Temp_C
  Constant29 : Constant  Value=BTMR_tiTempBase_C
  Constant30 : Constant  Value=BTMR_tiTempDebs_C
  Relational Operator20 : RelationalOperator  Operator=<=  OutDataTypeStr=boolean  RndMeth=Simplest
  BTMR_flgCoolChrgStage3ExtTemp : Outport
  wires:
  Relational Operator20/1 -> BMSDebounceStartZero/1
  BMSDebounceStartZero/1 -> BTMR_flgCoolChrgStage3ExtTemp/1
  BSPR_tCellTempMax/1 -> Relational Operator20/1
  Constant13/1 -> Relational Operator20/2
  Constant29/1 -> BMSDebounceStartZero/5, BMSDebounceStartZero/3
  Constant30/1 -> BMSDebounceStartZero/4, BMSDebounceStartZero/2

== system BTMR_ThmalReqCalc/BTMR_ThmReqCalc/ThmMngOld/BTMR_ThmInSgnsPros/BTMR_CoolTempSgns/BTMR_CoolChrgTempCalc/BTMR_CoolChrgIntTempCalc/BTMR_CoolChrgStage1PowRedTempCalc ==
  BSPR_tClntUsT : Inport
  BMSDebounceStartZero : AIWAYS_Powertrain_BMS_lib/Debounce & Delay/BMSDebounceStartZero
  Constant25 : Constant  Value=BTMR_t861CoolChrgIntLv2Temp_C
  Constant29 : Constant  Value=BTMR_tiTempBase_C
  Constant30 : Constant  Value=BTMR_tiTempDebs_C
  Relational Operator20 : RelationalOperator  Operator=<=  OutDataTypeStr=boolean  RndMeth=Simplest
  BTMR_flgCoolChrgStage1PowRedTemp : Outport
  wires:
  BSPR_tClntUsT/1 -> Relational Operator20/1
  BMSDebounceStartZero/1 -> BTMR_flgCoolChrgStage1PowRedTemp/1
  Relational Operator20/1 -> BMSDebounceStartZero/1
  Constant25/1 -> Relational Operator20/2
  Constant29/1 -> BMSDebounceStartZero/5, BMSDebounceStartZero/3
  Constant30/1 -> BMSDebounceStartZero/4, BMSDebounceStartZero/2

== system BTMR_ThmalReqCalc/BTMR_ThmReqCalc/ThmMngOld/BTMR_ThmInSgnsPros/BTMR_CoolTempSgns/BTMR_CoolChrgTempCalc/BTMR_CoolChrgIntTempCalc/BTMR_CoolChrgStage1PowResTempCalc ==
  BSPR_tClntUsT : Inport
  BMSDebounceStartZero : AIWAYS_Powertrain_BMS_lib/Debounce & Delay/BMSDebounceStartZero
  Constant25 : Constant  Value=BTMR_t861CoolChrgIntLv5Temp_C
  Constant29 : Constant  Value=BTMR_tiTempBase_C
  Constant30 : Constant  Value=BTMR_tiTempDebs_C
  Relational Operator20 : RelationalOperator  OutDataTypeStr=boolean  RndMeth=Simplest
  BTMR_flgCoolChrgStage1PowResTemp : Outport
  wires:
  Constant25/1 -> Relational Operator20/2
  Relational Operator20/1 -> BMSDebounceStartZero/1
  BMSDebounceStartZero/1 -> BTMR_flgCoolChrgStage1PowResTemp/1
  BSPR_tClntUsT/1 -> Relational Operator20/1
  Constant29/1 -> BMSDebounceStartZero/5, BMSDebounceStartZero/3
  Constant30/1 -> BMSDebounceStartZero/4, BMSDebounceStartZero/2

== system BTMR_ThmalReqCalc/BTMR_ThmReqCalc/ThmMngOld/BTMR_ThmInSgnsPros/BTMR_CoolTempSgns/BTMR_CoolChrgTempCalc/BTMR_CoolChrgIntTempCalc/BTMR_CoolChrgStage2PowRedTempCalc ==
  BSPR_tClntUsT : Inport
  BMSDebounceStartZero : AIWAYS_Powertrain_BMS_lib/Debounce & Delay/BMSDebounceStartZero
  Constant25 : Constant  Value=BTMR_t861CoolChrgIntLv1Temp_C
  Constant29 : Constant  Value=BTMR_tiTempBase_C
  Constant30 : Constant  Value=BTMR_tiTempDebs_C
  Relational Operator20 : RelationalOperator  Operator=<=  OutDataTypeStr=boolean  RndMeth=Simplest
  BTMR_flgCoolChrgStage2PowRedTemp : Outport
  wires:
  BSPR_tClntUsT/1 -> Relational Operator20/1
  BMSDebounceStartZero/1 -> BTMR_flgCoolChrgStage2PowRedTemp/1
  Relational Operator20/1 -> BMSDebounceStartZero/1
  Constant25/1 -> Relational Operator20/2
  Constant29/1 -> BMSDebounceStartZero/5, BMSDebounceStartZero/3
  Constant30/1 -> BMSDebounceStartZero/4, BMSDebounceStartZero/2

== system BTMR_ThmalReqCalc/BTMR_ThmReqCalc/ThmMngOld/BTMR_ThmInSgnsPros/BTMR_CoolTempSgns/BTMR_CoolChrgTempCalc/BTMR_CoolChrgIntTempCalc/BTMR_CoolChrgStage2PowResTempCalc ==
  BSPR_tClntUsT : Inport
  BMSDebounceStartZero : AIWAYS_Powertrain_BMS_lib/Debounce & Delay/BMSDebounceStartZero
  Constant25 : Constant  Value=BTMR_t861CoolChrgIntLv4Temp_C
  Constant29 : Constant  Value=BTMR_tiTempBase_C
  Constant30 : Constant  Value=BTMR_tiTempDebs_C
  Relational Operator20 : RelationalOperator  OutDataTypeStr=boolean  RndMeth=Simplest
  BTMR_flgCoolChrgStage2PowResTemp : Outport
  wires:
  Constant25/1 -> Relational Operator20/2
  Relational Operator20/1 -> BMSDebounceStartZero/1
  BMSDebounceStartZero/1 -> BTMR_flgCoolChrgStage2PowResTemp/1
  BSPR_tClntUsT/1 -> Relational Operator20/1
  Constant29/1 -> BMSDebounceStartZero/5, BMSDebounceStartZero/3
  Constant30/1 -> BMSDebounceStartZero/4, BMSDebounceStartZero/2

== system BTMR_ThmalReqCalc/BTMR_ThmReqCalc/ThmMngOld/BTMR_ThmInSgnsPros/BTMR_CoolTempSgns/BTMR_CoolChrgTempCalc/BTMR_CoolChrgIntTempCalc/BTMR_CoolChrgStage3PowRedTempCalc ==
  BSPR_tClntUsT : Inport
  BMSDebounceStartZero : AIWAYS_Powertrain_BMS_lib/Debounce & Delay/BMSDebounceStartZero
  Constant25 : Constant  Value=BTMR_t861CoolChrgIntLv0Temp_C
  Constant29 : Constant  Value=BTMR_tiTempBase_C
  Constant30 : Constant  Value=BTMR_tiTempDebs_C
  Relational Operator20 : RelationalOperator  Operator=<=  OutDataTypeStr=boolean  RndMeth=Simplest
  BTMR_flgCoolChrgStage3PowRedTemp : Outport
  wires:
  Constant25/1 -> Relational Operator20/2
  BMSDebounceStartZero/1 -> BTMR_flgCoolChrgStage3PowRedTemp/1
  BSPR_tClntUsT/1 -> Relational Operator20/1
  Constant29/1 -> BMSDebounceStartZero/5, BMSDebounceStartZero/3
  Constant30/1 -> BMSDebounceStartZero/4, BMSDebounceStartZero/2
  Relational Operator20/1 -> BMSDebounceStartZero/1

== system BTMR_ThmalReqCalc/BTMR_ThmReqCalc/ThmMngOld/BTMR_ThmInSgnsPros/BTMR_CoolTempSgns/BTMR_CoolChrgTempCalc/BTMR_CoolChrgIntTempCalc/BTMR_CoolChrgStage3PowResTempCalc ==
  BSPR_tClntUsT : Inport
  BMSDebounceStartZero : AIWAYS_Powertrain_BMS_lib/Debounce & Delay/BMSDebounceStartZero
  Constant25 : Constant  Value=BTMR_t861CoolChrgIntLv3Temp_C
  Constant29 : Constant  Value=BTMR_tiTempBase_C
  Constant30 : Constant  Value=BTMR_tiTempDebs_C
  Relational Operator20 : RelationalOperator  OutDataTypeStr=boolean  RndMeth=Simplest
  BTMR_flgCoolChrgStage3PowResTemp : Outport
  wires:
  BSPR_tClntUsT/1 -> Relational Operator20/1
  BMSDebounceStartZero/1 -> BTMR_flgCoolChrgStage3PowResTemp/1
  Relational Operator20/1 -> BMSDebounceStartZero/1
  Constant25/1 -> Relational Operator20/2
  Constant29/1 -> BMSDebounceStartZero/5, BMSDebounceStartZero/3
  Constant30/1 -> BMSDebounceStartZero/4, BMSDebounceStartZero/2

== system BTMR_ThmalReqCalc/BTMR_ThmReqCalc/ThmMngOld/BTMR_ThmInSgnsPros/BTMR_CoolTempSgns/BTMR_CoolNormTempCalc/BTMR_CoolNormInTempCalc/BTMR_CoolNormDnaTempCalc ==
  BSPR_tCellTempMax : Inport
  BMSDebounceStartZero : AIWAYS_Powertrain_BMS_lib/Debounce & Delay/BMSDebounceStartZero
  Constant13 : Constant  Value=BTMR_t861CoolNormExitTemp_C
  Constant29 : Constant  Value=BTMR_tiTempBase_C
  Constant30 : Constant  Value=BTMR_tiTempDebs_C
  Relational Operator20 : RelationalOperator  Operator=<=  OutDataTypeStr=boolean  RndMeth=Simplest
  BTMR_flgCoolNormDnaTemp : Outport
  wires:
  BSPR_tCellTempMax/1 -> Relational Operator20/1
  Constant13/1 -> Relational Operator20/2
  BMSDebounceStartZero/1 -> BTMR_flgCoolNormDnaTemp/1
  Relational Operator20/1 -> BMSDebounceStartZero/1
  Constant29/1 -> BMSDebounceStartZero/5, BMSDebounceStartZero/3
  Constant30/1 -> BMSDebounceStartZero/4, BMSDebounceStartZero/2

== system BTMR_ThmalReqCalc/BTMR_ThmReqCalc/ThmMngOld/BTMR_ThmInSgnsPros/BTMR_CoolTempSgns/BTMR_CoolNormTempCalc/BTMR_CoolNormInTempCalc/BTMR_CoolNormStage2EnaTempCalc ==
  BSPR_tCellTempMax : Inport
  BMSDebounceStartZero : AIWAYS_Powertrain_BMS_lib/Debounce & Delay/BMSDebounceStartZero
  Constant1 : Constant  Value=BTMR_t861CoolNormLv2Temp_C
  Constant29 : Constant  Value=BTMR_tiTempBase_C
  Constant30 : Constant  Value=BTMR_tiTempDebs_C
  Relational Operator20 : RelationalOperator  OutDataTypeStr=boolean  RndMeth=Simplest
  BTMR_flgCoolNormStage2EnaTemp : Outport
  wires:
  BSPR_tCellTempMax/1 -> Relational Operator20/1
  Constant1/1 -> Relational Operator20/2
  BMSDebounceStartZero/1 -> BTMR_flgCoolNormStage2EnaTemp/1
  Relational Operator20/1 -> BMSDebounceStartZero/1
  Constant29/1 -> BMSDebounceStartZero/5, BMSDebounceStartZero/3
  Constant30/1 -> BMSDebounceStartZero/4, BMSDebounceStartZero/2

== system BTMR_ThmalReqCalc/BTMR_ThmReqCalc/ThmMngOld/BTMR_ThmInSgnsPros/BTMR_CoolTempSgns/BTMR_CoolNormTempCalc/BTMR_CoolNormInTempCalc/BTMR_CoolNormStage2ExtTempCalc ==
  BSPR_tCellTempMax : Inport
  BMSDebounceStartZero : AIWAYS_Powertrain_BMS_lib/Debounce & Delay/BMSDebounceStartZero
  Constant13 : Constant  Value=BTMR_t861CoolNormExitLv2Temp_C
  Constant29 : Constant  Value=BTMR_tiTempBase_C
  Constant30 : Constant  Value=BTMR_tiTempDebs_C
  Relational Operator20 : RelationalOperator  Operator=<=  OutDataTypeStr=boolean  RndMeth=Simplest
  BTMR_flgCoolNormStage2ExtTemp : Outport
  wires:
  Relational Operator20/1 -> BMSDebounceStartZero/1
  BMSDebounceStartZero/1 -> BTMR_flgCoolNormStage2ExtTemp/1
  Constant13/1 -> Relational Operator20/2
  BSPR_tCellTempMax/1 -> Relational Operator20/1
  Constant29/1 -> BMSDebounceStartZero/5, BMSDebounceStartZero/3
  Constant30/1 -> BMSDebounceStartZero/4, BMSDebounceStartZero/2

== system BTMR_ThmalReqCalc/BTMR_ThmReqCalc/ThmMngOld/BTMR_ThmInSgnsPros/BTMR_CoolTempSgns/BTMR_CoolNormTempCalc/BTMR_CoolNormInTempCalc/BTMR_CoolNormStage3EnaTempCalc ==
  BSPR_tCellTempMax : Inport
  BMSDebounceStartZero : AIWAYS_Powertrain_BMS_lib/Debounce & Delay/BMSDebounceStartZero
  Constant1 : Constant  Value=BTMR_t861CoolNormLv3Temp_C
  Constant29 : Constant  Value=BTMR_tiTempBase_C
  Constant30 : Constant  Value=BTMR_tiTempDebs_C
  Relational Operator20 : RelationalOperator  OutDataTypeStr=boolean  RndMeth=Simplest
  BTMR_flgCoolNormStage3EnaTemp : Outport
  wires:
  Relational Operator20/1 -> BMSDebounceStartZero/1
  BMSDebounceStartZero/1 -> BTMR_flgCoolNormStage3EnaTemp/1
  Constant1/1 -> Relational Operator20/2
  BSPR_tCellTempMax/1 -> Relational Operator20/1
  Constant29/1 -> BMSDebounceStartZero/5, BMSDebounceStartZero/3
  Constant30/1 -> BMSDebounceStartZero/4, BMSDebounceStartZero/2

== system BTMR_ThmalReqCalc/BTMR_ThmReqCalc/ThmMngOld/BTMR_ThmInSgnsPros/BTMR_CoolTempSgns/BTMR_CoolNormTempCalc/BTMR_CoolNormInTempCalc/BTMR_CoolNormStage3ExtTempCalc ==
  BSPR_tCellTempMax : Inport
  BMSDebounceStartZero : AIWAYS_Powertrain_BMS_lib/Debounce & Delay/BMSDebounceStartZero
  Constant13 : Constant  Value=BTMR_t861CoolNormExitLv3Temp_C
  Constant29 : Constant  Value=BTMR_tiTempBase_C
  Constant30 : Constant  Value=BTMR_tiTempDebs_C
  Relational Operator20 : RelationalOperator  Operator=<=  OutDataTypeStr=boolean  RndMeth=Simplest
  BTMR_flgCoolNormStage3ExtTemp : Outport
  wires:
  BSPR_tCellTempMax/1 -> Relational Operator20/1
  Constant13/1 -> Relational Operator20/2
  BMSDebounceStartZero/1 -> BTMR_flgCoolNormStage3ExtTemp/1
  Relational Operator20/1 -> BMSDebounceStartZero/1
  Constant29/1 -> BMSDebounceStartZero/5, BMSDebounceStartZero/3
  Constant30/1 -> BMSDebounceStartZero/4, BMSDebounceStartZero/2

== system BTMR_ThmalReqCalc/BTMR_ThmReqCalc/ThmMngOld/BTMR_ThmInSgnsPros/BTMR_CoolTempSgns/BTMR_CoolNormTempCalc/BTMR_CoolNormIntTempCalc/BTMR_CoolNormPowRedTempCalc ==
  BSPR_tClntUsT : Inport
  BMSDebounceStartZero : AIWAYS_Powertrain_BMS_lib/Debounce & Delay/BMSDebounceStartZero
  Constant13 : Constant  Value=BTMR_t861CoolNormIntLv0Temp_C
  Constant29 : Constant  Value=BTMR_tiTempBase_C
  Constant30 : Constant  Value=BTMR_tiTempDebs_C
  Relational Operator20 : RelationalOperator  Operator=<=  OutDataTypeStr=boolean  RndMeth=Simplest
  BTMR_flgCoolNormPowRedTemp : Outport
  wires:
  Relational Operator20/1 -> BMSDebounceStartZero/1
  BMSDebounceStartZero/1 -> BTMR_flgCoolNormPowRedTemp/1
  Constant13/1 -> Relational Operator20/2
  BSPR_tClntUsT/1 -> Relational Operator20/1
  Constant29/1 -> BMSDebounceStartZero/5, BMSDebounceStartZero/3
  Constant30/1 -> BMSDebounceStartZero/4, BMSDebounceStartZero/2

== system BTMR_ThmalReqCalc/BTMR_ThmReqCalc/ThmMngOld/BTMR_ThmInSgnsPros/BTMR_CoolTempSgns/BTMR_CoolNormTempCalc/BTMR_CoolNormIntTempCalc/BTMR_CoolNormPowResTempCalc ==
  BSPR_tClntUsT : Inport
  BMSDebounceStartZero : AIWAYS_Powertrain_BMS_lib/Debounce & Delay/BMSDebounceStartZero
  Constant13 : Constant  Value=BTMR_t861CoolNormIntLv1Temp_C
  Constant29 : Constant  Value=BTMR_tiTempBase_C
  Constant30 : Constant  Value=BTMR_tiTempDebs_C
  Relational Operator20 : RelationalOperator  OutDataTypeStr=boolean  RndMeth=Simplest
  BTMR_flgCoolNormPowResTemp : Outport
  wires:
  BSPR_tClntUsT/1 -> Relational Operator20/1
  Constant13/1 -> Relational Operator20/2
  BMSDebounceStartZero/1 -> BTMR_flgCoolNormPowResTemp/1
  Relational Operator20/1 -> BMSDebounceStartZero/1
  Constant29/1 -> BMSDebounceStartZero/5, BMSDebounceStartZero/3
  Constant30/1 -> BMSDebounceStartZero/4, BMSDebounceStartZero/2

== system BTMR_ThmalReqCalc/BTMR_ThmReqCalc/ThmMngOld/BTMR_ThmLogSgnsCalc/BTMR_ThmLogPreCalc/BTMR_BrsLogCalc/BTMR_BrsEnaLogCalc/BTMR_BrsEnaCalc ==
  BTMR_flgBrsInLogSgns : Inport
  Bus Selector : BusSelector  OutputSignals=BTMR_flgBrsDCLogSgns,BTMR_flgBrsACLogSgns,BTMR_flgBrsDrvLogSgns
  Bus Selector1 : BusSelector  OutputSignals=BTMR_flgBrsIntEna1
  Bus Selector2 : BusSelector  OutputSignals=BTMR_flgBrsIntEna2
  Bus Selector3 : BusSelector  OutputSignals=BTMR_flgBrsIntEna3
  Logical Operator3 : Logic  Operator=OR  Inputs=3  AllPortsSameDT=off  OutDataTypeStr=boolean
  BTMR_flgBrsEna : Outport
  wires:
  BTMR_flgBrsInLogSgns/1 -> Bus Selector/1
  Bus Selector/1 -> Bus Selector1/1  "<BTMR_flgBrsDCLogSgns>"
  Bus Selector/3 -> Bus Selector3/1  "<BTMR_flgBrsDrvLogSgns>"
  Logical Operator3/1 -> BTMR_flgBrsEna/1  "BTMR_flgBrsEna"
  Bus Selector1/1 -> Logical Operator3/1  "<BTMR_flgBrsIntEna1>"
  Bus Selector3/1 -> Logical Operator3/3  "<BTMR_flgBrsIntEna3>"
  Bus Selector2/1 -> Logical Operator3/2  "<BTMR_flgBrsIntEna2>"
  Bus Selector/2 -> Bus Selector2/1  "<BTMR_flgBrsACLogSgns>"

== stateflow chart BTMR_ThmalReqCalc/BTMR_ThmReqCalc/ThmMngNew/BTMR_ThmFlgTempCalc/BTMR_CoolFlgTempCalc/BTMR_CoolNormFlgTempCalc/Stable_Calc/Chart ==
  state Default_Stt
    en:
    i=uint8(0);
    flg_out=false;
  state AddCourse_Stt
    en:
    flg_out=true;
    du:
    i = i + uint8(1);
  (default) -> Default_Stt
  AddCourse_Stt -> Default_Stt : [ i>cntStable ]
  Default_Stt -> AddCourse_Stt : [ trigger_in==true ]
  data: i local uint8; trigger_in input boolean; flg_out output boolean; cntStable input

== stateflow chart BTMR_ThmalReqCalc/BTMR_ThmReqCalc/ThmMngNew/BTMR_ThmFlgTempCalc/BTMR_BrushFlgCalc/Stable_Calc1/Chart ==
  state Default_Stt
    en:
    i=uint8(0);
    flg_out=false;
  state AddCourse_Stt
    en:
    flg_out=true;
    du:
    i = i + uint8(1);
  (default) -> Default_Stt
  AddCourse_Stt -> Default_Stt : [ i>cntStable ]
  Default_Stt -> AddCourse_Stt : [ trigger_in==true ]
  data: i local uint8; trigger_in input boolean; flg_out output boolean; cntStable input

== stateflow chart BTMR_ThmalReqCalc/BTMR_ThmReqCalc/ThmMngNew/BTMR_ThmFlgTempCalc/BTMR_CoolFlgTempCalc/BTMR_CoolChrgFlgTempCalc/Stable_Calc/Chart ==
  state Default_Stt
    en:
    i=uint8(0);
    flg_out=false;
  state AddCourse_Stt
    en:
    flg_out=true;
    du:
    i = i + uint8(1);
  (default) -> Default_Stt
  AddCourse_Stt -> Default_Stt : [ i>cntStable ]
  Default_Stt -> AddCourse_Stt : [ trigger_in==true ]
  data: i local uint8; trigger_in input boolean; flg_out output boolean; cntStable input

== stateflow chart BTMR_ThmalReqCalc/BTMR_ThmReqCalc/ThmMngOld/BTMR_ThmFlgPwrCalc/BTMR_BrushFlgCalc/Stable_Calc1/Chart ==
  state Default_Stt
    en:
    i=uint8(0);
    flg_out=false;
  state AddCourse_Stt
    en:
    flg_out=true;
    du:
    i = i + uint8(1);
  (default) -> Default_Stt
  AddCourse_Stt -> Default_Stt : [ i>cntStable ]
  Default_Stt -> AddCourse_Stt : [ trigger_in==true ]
  data: i local uint8; trigger_in input boolean; flg_out output boolean; cntStable input

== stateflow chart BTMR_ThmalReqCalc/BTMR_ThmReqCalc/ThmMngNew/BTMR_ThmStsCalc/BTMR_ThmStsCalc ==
  state Default_Stt
    en:
    stHtgSts=enmThmHeatSts.InActive;
    stCoolSts=enmThmCoolSts.InActive;
    stBrsSts=enmThmBrsSts.INACTIVE;
  state HtgDC_Stt
    en:
    stHtgSts=enmThmHeatSts.HeatDC;
    stCoolSts=enmThmCoolSts.InActive;
    stBrsSts=enmThmBrsSts.INACTIVE;
  state Standby_Stt
    en:
    Local_DebCnt=uint16(0);
    stHtgSts=enmThmHeatSts.InActive;
    stCoolSts=enmThmCoolSts.InActive;
    stBrsSts=enmThmBrsSts.INACTIVE;
    du:
    (default) -> (junction 130)
    Standby_Stt -> (junction 130)
    (junction 130) -> (junction 134) : [Local_DebCnt<=uint16(600)]
    (junction 130) -> (junction 157) : {Local_DebCnt=uint16(600);}
    (junction 134) -> (junction 152) : {Local_DebCnt++;}
    (junction 152) -> (junction 157)
    (junction 157) -> (junction 147)
  state CoolChrg_Stt
    en:
    stHtgSts=enmThmHeatSts.InActive;
    stCoolSts=enmThmCoolSts.CoolChrg;
    stBrsSts=enmThmBrsSts.INACTIVE;
  state HtgAC_Stt
    en:
    stHtgSts=enmThmHeatSts.HeatAC;
    stCoolSts=enmThmCoolSts.InActive;
    stBrsSts=enmThmBrsSts.INACTIVE;
  state CoolNorm_Stt
    en:
    stHtgSts=enmThmHeatSts.InActive;
    stCoolSts=enmThmCoolSts.CoolNorm;
    stBrsSts=enmThmBrsSts.INACTIVE;
  state HtgDrv_Stt
    en:
    stHtgSts=enmThmHeatSts.HeatDrv;
    stCoolSts=enmThmCoolSts.InActive;
    stBrsSts=enmThmBrsSts.INACTIVE;
  state Brush_Stt
    en:
    stHtgSts=enmThmHeatSts.InActive;
    stCoolSts=enmThmCoolSts.InActive;
    stBrsSts=enmThmBrsSts.ACTIVE;
  (default) -> Default_Stt
  Default_Stt -> Standby_Stt
  Standby_Stt -> HtgDC_Stt : [ HtgDCEna &&...  (HtgDCThmEnd==false)&&... Local_DebCnt>=uint16(600) ]
  Standby_Stt -> CoolChrg_Stt : [ CoolChrgEna &&...  (CoolChrgThmEnd==false)&&... Local_DebCnt>=uint16(600) ]
  HtgDC_Stt -> Standby_Stt : [ HtgDCThmEnd... || HtgDCDna ]
  CoolChrg_Stt -> Standby_Stt : [ CoolChrgThmEnd... || CoolChrgDna ]
  Standby_Stt -> HtgAC_Stt : [ HtgACEna &&...  (HtgACThmEnd==false)&&... Local_DebCnt>=uint16(600) ]
  HtgAC_Stt -> Standby_Stt : [ HtgACThmEnd... || HtgACDna ]
  Standby_Stt -> CoolNorm_Stt : [ CoolNormEna &&...  (CoolNormThmEnd==false)&&... Local_DebCnt>=uint16(600) ]
  Standby_Stt -> HtgDrv_Stt : [ HtgDrvEna &&...  (HtgDrvThmEnd==false)&&... Local_DebCnt>=uint16(600) ]
  CoolNorm_Stt -> Standby_Stt : [ CoolNormThmEnd...  || CoolNormDna ]
  HtgDrv_Stt -> Standby_Stt : [ HtgDrvThmEnd... || HtgDrvDna ]
  Standby_Stt -> Brush_Stt : [ (BrsEna && BrsStart) &&... (BrsThmEnd==false)&&... Local_DebCnt>=uint16(600)]
  Brush_Stt -> Standby_Stt : [ (BrsEna==false) ||...  (BrsThmEnd || BrsDna) ]
  data: stBrsSts output Enum: enmThmBrsSts; BrsEna input; HtgDCEna input; HtgACEna input; HtgDrvEna input; CoolNormEna input; CoolChrgEna input; BrsDna input; HtgDCDna input; HtgACDna input; HtgDrvDna input; CoolNormDna input; CoolChrgDna input; BrsThmEnd input; stHtgSts output Enum: enmThmHeatSts; stCoolSts output Enum: enmThmCoolSts; HtgDCThmEnd input; HtgACThmEnd input; HtgDrvThmEnd input; CoolNormThmEnd input; CoolChrgThmEnd input; BrsStart input; Local_DebCnt local uint16

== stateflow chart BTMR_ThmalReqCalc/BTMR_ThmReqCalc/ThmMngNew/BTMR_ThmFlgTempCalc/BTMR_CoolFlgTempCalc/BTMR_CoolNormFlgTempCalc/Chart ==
  state CoolNormDefault
    en:
    BTMR_stsClntStg=enmThmCoolNormStg_891.Default;
  state CoolNormStage1
    en:
    BTMR_stsClntStg=enmThmCoolNormStg_891.Stg_Lv1;
  state CoolNormStage2
    en:
    BTMR_stsClntStg=enmThmCoolNormStg_891.Stg_Lv2;
  state CoolNormStage3
    en:
    BTMR_stsClntStg=enmThmCoolNormStg_891.Stg_Lv3;
  (default) -> CoolNormDefault
  CoolNormDefault -> CoolNormStage1
  CoolNormStage2 -> CoolNormStage1 : [ CoolNormStage2Ext ]
  CoolNormStage1 -> CoolNormStage2 : [ CoolNormStage2Ena ]
  CoolNormStage3 -> CoolNormStage2 : [ CoolNormStage3Ext ]
  CoolNormStage2 -> CoolNormStage3 : [ CoolNormStage3Ena ]
  data: CoolNormStage2Ena input; CoolNormStage3Ena input; BTMR_stsClntStg output Enum: enmThmCoolNormStg_891; CoolNormStage2Ext input; CoolNormStage3Ext input

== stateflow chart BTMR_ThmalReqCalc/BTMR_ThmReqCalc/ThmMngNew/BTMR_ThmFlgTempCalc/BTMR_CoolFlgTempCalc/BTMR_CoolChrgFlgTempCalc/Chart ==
  state CoolChrgDefault
    en:
    BTMR_stsClntStg=enmThmCoolChrgStg_891.Default;
  state CoolChrgStage1
    en:
    BTMR_stsClntStg=enmThmCoolChrgStg_891.Stg_Lv1;
  state CoolChrgStage2
    en:
    BTMR_stsClntStg=enmThmCoolChrgStg_891.Stg_Lv2;
  state CoolChrgStage3
    en:
    BTMR_stsClntStg=enmThmCoolChrgStg_891.Stg_Lv3;
  (default) -> CoolChrgDefault
  CoolChrgDefault -> CoolChrgStage1
  CoolChrgStage2 -> CoolChrgStage1 : [ CoolChrgStage2Ext ]
  CoolChrgStage1 -> CoolChrgStage2 : [ CoolChrgStage2Ena ]
  CoolChrgStage3 -> CoolChrgStage2 : [ CoolChrgStage3Ext ]
  CoolChrgStage2 -> CoolChrgStage3 : [ CoolChrgStage3Ena ]
  data: CoolChrgStage2Ena input; CoolChrgStage3Ena input; BTMR_stsClntStg output Enum: enmThmCoolChrgStg_891; CoolChrgStage2Ext input; CoolChrgStage3Ext input
